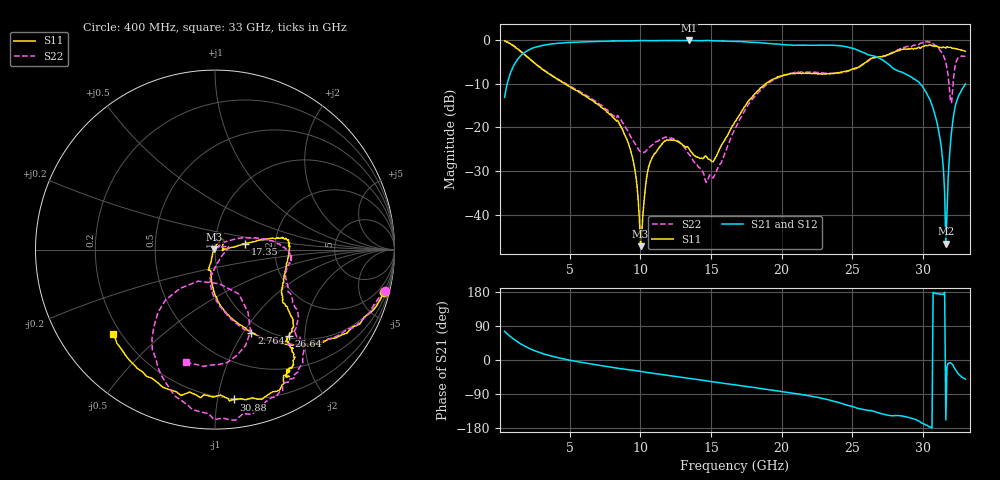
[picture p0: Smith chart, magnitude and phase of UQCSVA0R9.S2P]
!  Part Number UQCSVA0R9  Mounting Orientation: Horizontal
!  Description: Ultra Low ESR Microwave capacitors
!  Application: Coupling, Bypass, Tuning, DC Block
!  Filters, Matching
# GHZ S DB R 50
! Freq  |S11|  S11 Ph  |S21|  S21 Ph  |S12|  S12 Ph  |S22|  S22 Ph
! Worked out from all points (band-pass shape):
!   401 points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, 400 MHz to 33 GHz, reference 50 ohm
!   highest |S21| = -0.15 dB at 13.44 GHz (marker M1); lowest = -46.6 dB at 31.61 GHz (marker M2)
!   |S21| within 3 dB of the highest: 1.713 GHz to 25.96 GHz (24.25 GHz wide, 175 % of centre)
!   lowest |S11| = -47.1 dB at 10.02 GHz (marker M3), VSWR 1.01, Z = 49.6 + j0.11 ohm
!   |S11| at or under -10 dB: 4.634 GHz to 18.89 GHz (14.26 GHz wide, 121 % of centre)
!   |S22| runs from -32.6 to -0.2 dB; largest |S21 - S12| = 0.0084
!   S11 on the Smith chart (normalised r, x): 400 MHz: 0.94, -7.95; 2.764 GHz: 0.88, -1.09; 17.35 GHz: 1.40, +0.10; 26.64 GHz: 1.04, -1.67; 30.88 GHz: 0.19, -1.11; 33 GHz: 0.17, -0.35
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0.4  -0.25 -14.2  -13.14 75.5  -13.16 75.4  -0.24 -13.7
1.378  -2.23 -42.5  -4.23 46.6  -4.20 46.6  -2.19 -41.7
2.764  -5.94 -66.4  -1.52 21.1  -1.52 21.1  -5.93 -66.3
5.861  -12.35 -90.9  -0.49 -6.4  -0.49 -6.5  -12.07 -92.8
8.876  -21.55 -108.5  -0.26 -24.1  -0.27 -24.1  -19.53 -91.5
9.528  -28.08 -113.5  -0.23 -27.4  -0.25 -27.5  -23.22 -73.9
10.017  -47.14 165.4  -0.16 -30.1  -0.16 -30.3  -25.51 -48.9
10.588  -29.07 66.6  -0.22 -33.5  -0.22 -33.5  -24.63 -14.6
11.321  -24.71 60.5  -0.19 -37.1  -0.21 -37.2  -22.95 5.0
13.44  -24.85 35.5  -0.15 -48.6  -0.17 -48.6  -26.12 18.2
15.152  -27.86 -2.8  -0.24 -57.8  -0.23 -57.8  -31.56 40.2
16.7  -18.72 8.8  -0.35 -65.6  -0.35 -65.4  -20.35 31.6
17.352  -15.39 11.5  -0.45 -69.1  -0.44 -69.1  -16.42 24.4
22.161  -7.73 -3.0  -1.25 -95.9  -1.23 -95.7  -7.40 -8.1
26.643  -3.98 -49.3  -3.78 -137.0  -3.79 -136.5  -4.04 -43.2
27.621  -3.21 -52.4  -5.73 -146.4  -5.74 -146.1  -3.34 -45.9
29.496  -2.02 -58.8  -9.21 -157.0  -9.15 -157.3  -1.11 -66.8
30.881  -1.50 -82.9  -17.56 175.4  -17.56 176.2  -1.32 -102.9
31.615  -1.87 -100.1  -46.57 -158.2  -45.97 -153.8  -5.19 -128.3
31.941  -1.72 -110.7  -23.76 -7.6  -23.77 -8.2  -14.00 -118.3
32.185  -1.91 -118.4  -16.88 -18.8  -16.88 -18.7  -8.10 -62.1
33  -2.62 -140.3  -10.11 -50.5  -10.05 -50.7  -3.82 -104.5
